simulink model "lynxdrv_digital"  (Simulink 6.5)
settings: Solver=FixedStepDiscrete  StartTime=0.0  StopTime=5  FixedStep=1/WorkFreq  RelTol=1e-3
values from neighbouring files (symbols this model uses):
  IPAddrStr = '192.168.1.34'    [Dados_AC1160.m]
  WorkFreq = 200    [Dados_AC1160.m]
undefined symbols (not defined in the file or in its folder): HRPCFreqCal

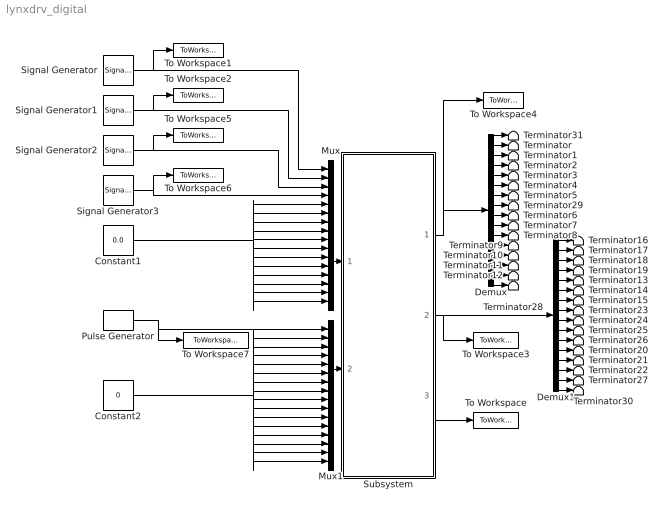
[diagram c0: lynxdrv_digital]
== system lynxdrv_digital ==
  Constant1 : Constant  Value=0.0  OutDataType=sfix(16)  ConRadixGroup=Use specified scaling  OutScaling=2^0  SampleTime=inf  FramePeriod=inf
  Constant2 : Constant  Value=0  OutDataType=sfix(16)  ConRadixGroup=Use specified scaling  OutScaling=2^0  SampleTime=inf  FramePeriod=inf
  Demux : Demux  Outputs=16
  Demux1 : Demux  Outputs=16
  Mux : Mux  Inputs=16
  Mux1 : Mux  Inputs=16
  Pulse Generator : DiscretePulseGenerator  PulseType=Time based  Period=1  PulseWidth=50
  Signal Generator : SignalGenerator  Amplitude=5
  Signal Generator1 : SignalGenerator  WaveForm=sawtooth  Amplitude=5
  Signal Generator2 : SignalGenerator  WaveForm=square  Amplitude=5  Frequency=3
  Signal Generator3 : SignalGenerator  Amplitude=5  Frequency=2
  Subsystem : Subsystem  mask{IPAddrStr=IPAddrStr, BaseFreq=4000, WorkFreq=WorkFreq, CalFreq=HRPCFreqCal(2), RangeIdx=-10V .. +10V}
      mask prompts: IPAddrStr "Endereço IP módulo Lynx"; BaseFreq "Frequência base do módulo Lynx"; WorkFreq "Frequência de amostragem"; CalFreq "Frequência calibrada do TSC"; RangeIdx "Range"
  Terminator{,1..31} (32 alike) : Terminator
  To Workspace : ToWorkspace  VariableName=status  SampleTime=-1  SaveFormat=Array
  To Workspace1 : ToWorkspace  VariableName=entrada1  SampleTime=1/WorkFreq  SaveFormat=Array
  To Workspace2 : ToWorkspace  VariableName=entrada2  SampleTime=1/WorkFreq  SaveFormat=Array
  To Workspace3 : ToWorkspace  VariableName=outdig  SampleTime=-1  SaveFormat=Array
  To Workspace4 : ToWorkspace  VariableName=out  SampleTime=1/WorkFreq  SaveFormat=Array
  To Workspace5 : ToWorkspace  VariableName=entrada3  SampleTime=1/WorkFreq  SaveFormat=Array
  To Workspace6 : ToWorkspace  VariableName=entrada4  SampleTime=1/WorkFreq  SaveFormat=Array
  To Workspace7 : ToWorkspace  VariableName=entrada_dig  SampleTime=1/WorkFreq  SaveFormat=Array
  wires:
  Mux/1 -> Subsystem/1(In1)
  Mux1/1 -> Subsystem/2(In2)
  Subsystem/1(Out1) -> Demux/1, To Workspace4/1
  Subsystem/2(Out2) -> To Workspace3/1, Demux1/1
  Subsystem/3(Out3) -> To Workspace/1
  Constant1/1 -> Mux/5, Mux/6, Mux/7, Mux/8, Mux/14, Mux/15, Mux/16, Mux/13, Mux/12, Mux/11, Mux/10, Mux/9
  Demux/2 -> Terminator/1
  Demux/3 -> Terminator1/1
  Demux/15 -> Terminator12/1
  Demux/14 -> Terminator11/1
  Demux/13 -> Terminator10/1
  Demux/12 -> Terminator9/1
  Demux/11 -> Terminator8/1
  Demux/10 -> Terminator7/1
  Demux/9 -> Terminator6/1
  Demux/7 -> Terminator5/1
  Demux/6 -> Terminator4/1
  Demux/5 -> Terminator3/1
  Demux/4 -> Terminator2/1
  Demux1/2 -> Terminator17/1
  Demux1/3 -> Terminator18/1
  Demux1/4 -> Terminator19/1
  Demux1/5 -> Terminator13/1
  Demux1/6 -> Terminator14/1
  Demux1/8 -> Terminator23/1
  Demux1/9 -> Terminator24/1
  Demux1/10 -> Terminator25/1
  Demux1/11 -> Terminator26/1
  Demux1/12 -> Terminator20/1
  Demux1/13 -> Terminator21/1
  Demux1/14 -> Terminator22/1
  Demux1/15 -> Terminator27/1
  Demux1/7 -> Terminator15/1
  Demux/16 -> Terminator28/1
  Demux/8 -> Terminator29/1
  Demux1/16 -> Terminator30/1
  Demux/1 -> Terminator31/1
  Pulse Generator/1 -> Mux1/1, To Workspace7/1
  Constant2/1 -> Mux1/2, Mux1/3, Mux1/4, Mux1/5, Mux1/6, Mux1/7, Mux1/8, Mux1/9, Mux1/10, Mux1/11, Mux1/12, Mux1/13, Mux1/14, Mux1/15, Mux1/16
  Demux1/1 -> Terminator16/1
  Signal Generator/1 -> Mux/1, To Workspace1/1
  Signal Generator3/1 -> Mux/4, To Workspace6/1
  Signal Generator2/1 -> Mux/3, To Workspace5/1
  Signal Generator1/1 -> Mux/2, To Workspace2/1

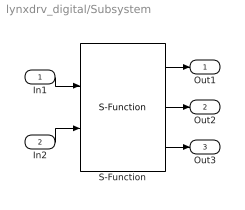
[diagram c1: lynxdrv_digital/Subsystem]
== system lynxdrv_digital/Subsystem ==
  In1 : Inport
  In2 : Inport  Port=2
  S-Function : S-Function  FunctionName=Sfcn_UDPdrv  Parameters=IPAddrStr,WorkFreq,CalFreq,RangeIdx,BaseFreq
  Out1 : Outport
  Out2 : Outport  Port=2
  Out3 : Outport  Port=3
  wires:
  S-Function/1 -> Out1/1
  In1/1 -> S-Function/1
  S-Function/2 -> Out2/1
  In2/1 -> S-Function/2
  S-Function/3 -> Out3/1
